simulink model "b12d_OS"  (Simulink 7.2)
settings: Solver=ode3  SolverMode=SingleTasking  StartTime=0.0  StopTime=0.2  FixedStep=10e-6  MaxStep=1e-5  RelTol=1e-3  AbsTol=1e-3

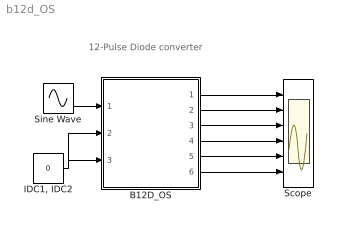
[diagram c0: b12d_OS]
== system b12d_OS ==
  note: 12-Pulse Diode converter
  B12D_OS : Subsystem  mask{LS=1e-4, nyy=1, nyd=sqrt(3), LT=1e-4, LD=1e-3, ILD0=200, C=1e-3, VC0=600, RL=2}
      mask prompts: LS "Source Inductance"; nyy "Trafo YY turns Ratio"; nyd "Trafo YD turns Ratio"; LT "Transformer Inductance"; LD "DC Inductance"; ILD0 "Initial Current ILD0"; C "Load Capacitance"; VC0 "Initial Cap Voltage"; RL "Load Resistance"
      mask help: 12-Pulse Diode Bridge Converter Input Vector u: u[0]= Vs1.v u[1]= Vs2.v u[2]= Vs3.v u[3]= IDC1.i u[4]= IDC2.i Output Vector y: y[0]= D11.I y[1]= D11.V y[2]= D12.I y[3]= D12.V y[4]= Lc1.I y[5]= Lc2.I y[6]= Lc3.I y[7]= Ld1.I y[8]= Ld2.I y[9]= VDC1.V y[10]= VDC2.V y[11]= VC1.V y[12]= VC2.V Parameter Vector p: p[0]= Lc1.L p[0]= Lc2.L p[0]= Lc3.L p[1]= nyy p[2]= nyd p[3]= LT.L p[4]= Ld.L p[5]= Ld.IL0 p[6]= C1.C p[7]= C1.vC0 p[8]= R1.r You can pause the simulation during running, change the Parameters you want and continue the Simulation
  "IDC1, IDC2" : Constant  Value=0  OutDataType=sfix(16)  OutScaling=2^0
  Scope : Scope  NumInputPorts=6
  Sine Wave : Sin  Amplitude=230*sqrt(2)  Frequency=2*pi*50  Phase="[0  -2*pi/3  -4*pi/3]"  SampleTime=0
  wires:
  Sine Wave/1 -> B12D_OS/1(vS)
  "IDC1, IDC2"/1 -> B12D_OS/3(iDC2), B12D_OS/2(iDC1)
  B12D_OS/1("iD1, vD1") -> Scope/1
  B12D_OS/2("iD2, vD2") -> Scope/2
  B12D_OS/3("iLc1, iLc2, iLc3") -> Scope/3
  B12D_OS/6(vC1,vC2) -> Scope/6
  B12D_OS/4(iLd1,iLd2) -> Scope/4
  B12D_OS/5(vDC1,vDC2) -> Scope/5

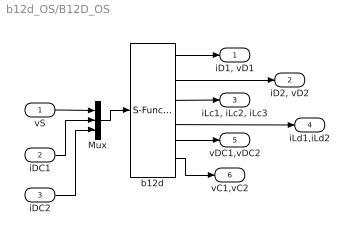
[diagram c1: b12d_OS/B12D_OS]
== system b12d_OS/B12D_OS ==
  vS : Inport  OutDataType=sfix(16)  OutScaling=2^0
  iDC1 : Inport  Port=2  OutDataType=sfix(16)  OutScaling=2^0
  iDC2 : Inport  Port=3  OutDataType=sfix(16)  OutScaling=2^0
  Mux : Mux  Inputs="[3  1  1]"
  b12d : S-Function  FunctionName=s_b12d_OS  Parameters="[ LS  nyy  nyd   LT  LD ILD0 C  VC0  RL]"  EnableBusSupport=off
  "iD1, vD1" : Outport  OutDataType=sfix(16)  OutScaling=2^0
  "iD2, vD2" : Outport  Port=2  OutDataType=sfix(16)  OutScaling=2^0
  "iLc1, iLc2, iLc3" : Outport  Port=3  OutDataType=sfix(16)  OutScaling=2^0
  iLd1,iLd2 : Outport  Port=4  OutDataType=sfix(16)  OutScaling=2^0
  vDC1,vDC2 : Outport  Port=5  OutDataType=sfix(16)  OutScaling=2^0
  vC1,vC2 : Outport  Port=6  OutDataType=sfix(16)  OutScaling=2^0
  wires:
  b12d/4 -> iLd1,iLd2/1
  Mux/1 -> b12d/1
  iDC1/1 -> Mux/2
  vS/1 -> Mux/1
  b12d/2 -> "iD2, vD2"/1
  b12d/1 -> "iD1, vD1"/1
  b12d/3 -> "iLc1, iLc2, iLc3"/1
  iDC2/1 -> Mux/3
  b12d/5 -> vDC1,vDC2/1
  b12d/6 -> vC1,vC2/1
